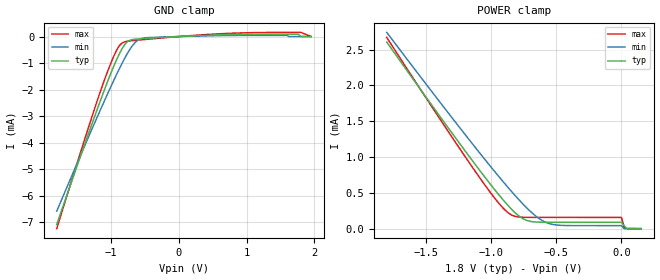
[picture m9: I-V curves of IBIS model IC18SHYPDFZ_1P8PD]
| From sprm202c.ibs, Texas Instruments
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|   Model IC18SHYPDFZ_1P8PD
[Model]   IC18SHYPDFZ_1P8PD
Model_type   Input
Polarity   Non-Inverting
Vinl =   0.8400V
Vinh =   0.9800V
C_comp   0.8000pF   0.9300pF   0.6600pF
[Model Spec]
|   typ   min   max
Vinh   0.98V   0.86V   1.05V
Vinl   0.84V   0.70V   0.91V
[Temperature Range]   25.0000   0.1250k   -40.0000
[Voltage Range]   1.8000V   1.6200V   1.9500V
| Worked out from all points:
|   GND clamp passes 1 mA (typ) near -0.94 V on its own axis
|   POWER clamp passes 1 mA (typ) near -1.16 V on its own axis
[GND_clamp]
| voltage   I(typ)   I(min)   I(max)
-1.8V     -7.089mA   -6.589mA   -7.249mA
-1.4V     -4.155mA   -4.193mA   -3.975mA
-1.12V    -2.169mA   -2.558mA   -1.802mA
-960mV    -1.123mA   -1.66mA    -749.1uA
-840mV    -473.4uA   -1.028mA   -249.1uA
-760mV    -199.9uA   -646.7uA   -178.8uA
-680mV    -113.1uA   -331.5uA   -154.2uA
-520mV    -77.82uA   -58.23uA   -115.9uA
1.08V     85.54uA    41.28uA    146.4uA
1.76V     88.59uA    0A         156.1uA
1.8V      0A         0A         156.2uA
1.95V     0A         0A         0A
[POWER_clamp]
| voltage   I(typ)   I(min)   I(max)
-1.8V     2.606mA    2.741mA    2.671mA
-1.12V    893.2uA    1.132mA    797.1uA
-960mV    517uA      770.9uA    398.3uA
-860mV    303.9uA    554.6uA    209.6uA
-740mV    124.8uA    314.7uA    158.6uA
-640mV    91.39uA    152uA      157.7uA
-560mV    89.35uA    74.38uA    157.6uA
-440mV    89.11uA    44.5uA     157.4uA
0V        88.64uA    41.95uA    156.6uA
20mV      44.32uA    0A         20.8uA
40mV      0A         0A         3.2uA
150mV     0A         0A         0A
